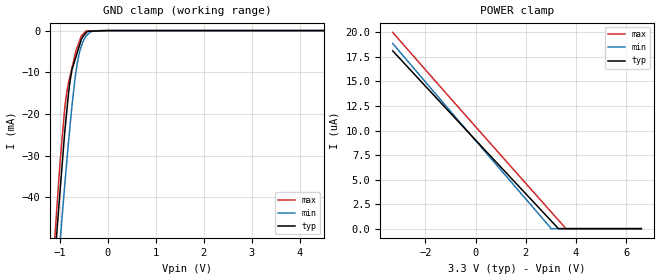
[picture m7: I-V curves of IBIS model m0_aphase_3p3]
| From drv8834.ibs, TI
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|   m0_aphase_3p3 Model
[Model]   m0_aphase_3p3
Model_type   Input
Vinl = 0.7
Vinh = 2
|   typ   min   max
|   (nom PVT)   (fast PVT)   (slow PVT)
|C_comp from frequency sweep method (F=250KHz)
|Average
|C_comp   3.006e-12   2.785e-12   3.226e-12
|C_comp from LC tank measurement(L=1nH)
|Average
|Resonant Frequency(Hz)   4.340e+09   4.370e+09   4.270e+09
 C_comp   1.346e-12   1.328e-12   1.391e-12
| Where nom  PVT is Nominal Process, 3.3V, 27C
|   Fast PVT is Strong Process,  3.6V, -40C
|   Slow PVT is Weak Process,   3V, 125C
[Voltage Range]   3.3   3   3.6
|Ambient Temperature   25   150   -40
|Junction Temperature
[Temperature Range]   27   125   -40
[Power Clamp Reference]   3.3   3   3.6
[GND Clamp Reference]   0   0   0
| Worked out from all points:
|   GND clamp passes 1 mA (typ) near -0.49 V on its own axis
[GND Clamp]
|   Voltage   I(typ)   I(min)   I(max)
-3.3V     -460.7mA   -437.6mA   -483mA
-1.166V   -65.08mA   -75.53mA   -59.75mA
-1.065V   -48.71mA   -60.47mA   -42.9mA
-1.001V   -39.18mA   -51.41mA   -32.24mA
-896.4mV  -24.04mA   -36.69mA   -18.29mA
-782.1mV  -11.67mA   -22.16mA   -10.59mA
-690mV    -7.215mA   -12.1mA    -6.104mA
-633mV    -5.107mA   -7.54mA    -3.838mA
-531mV    -1.658mA   -2.971mA   -1.021mA
-453.6mV  -537.6uA   -1.305mA   -112.2uA
-3mV      0A         -18.76nA   0A
6.6V      0A         0A         0A
[POWER Clamp]
|   Voltage   I(typ)   I(min)   I(max)
-3.3V     18.13uA    18.87uA    20uA
2.997V    828.3nA    0A         1.739uA
3.297V    0A         0A         874.5nA
3.604V    0A         0A         0A
6.6V      0A         0A         0A
